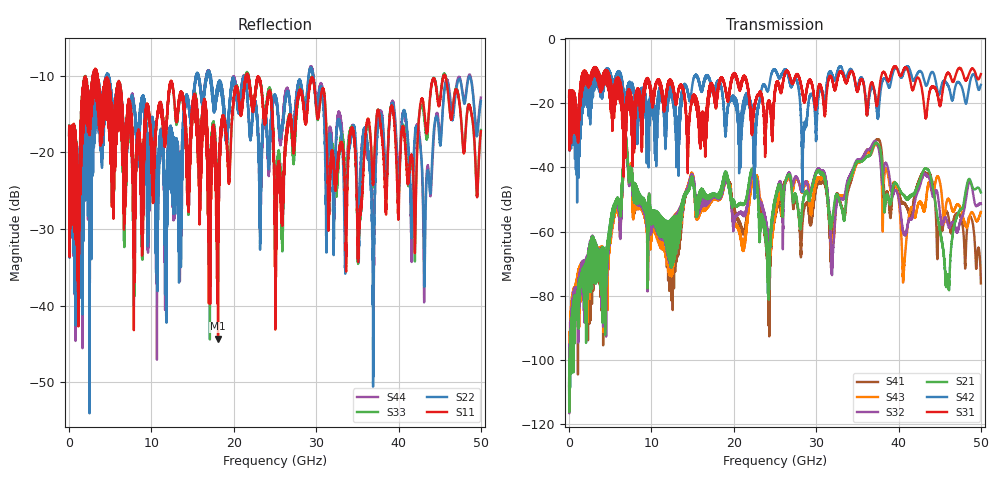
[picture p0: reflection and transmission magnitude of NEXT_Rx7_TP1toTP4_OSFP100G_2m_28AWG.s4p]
! Touchstone data
! Created: 27-Feb-2019 by IdEM 12 (12.1.0)
! COMMENTS
!  Created Wed Feb 27 12:03:36 2019
!  64 Port Network Data from SP1.SP block
!  freq  magS1_1  angS1_1  magS1_2  angS1_2  magS1_3  angS1_3  magS1_4  angS1_4
!  magS1_5  angS1_5  magS1_6  angS1_6  magS1_7  angS1_7  magS1_8  angS1_8
!  magS1_9  angS1_9  magS1_10  angS1_10  magS1_11  angS1_11  magS1_12  angS1_12
!  magS1_13  angS1_13  magS1_14  angS1_14  magS1_15  angS1_15  magS1_16  angS1_16
!  magS1_17  angS1_17  magS1_18  angS1_18  magS1_19  angS1_19  magS1_20  angS1_20
!  magS1_21  angS1_21  magS1_22  angS1_22  magS1_23  angS1_23  magS1_24  angS1_24
!  magS1_25  angS1_25  magS1_26  angS1_26  magS1_27  angS1_27  magS1_28  angS1_28
!  magS1_29  angS1_29  magS1_30  angS1_30  magS1_31  angS1_31  magS1_32  angS1_32
!  magS1_33  angS1_33  magS1_34  angS1_34  magS1_35  angS1_35  magS1_36  angS1_36
!  magS1_37  angS1_37  magS1_38  angS1_38  magS1_39  angS1_39  magS1_40  angS1_40
!  magS1_41  angS1_41  magS1_42  angS1_42  magS1_43  angS1_43  magS1_44  angS1_44
!  magS1_45  angS1_45  magS1_46  angS1_46  magS1_47  angS1_47  magS1_48  angS1_48
!  magS1_49  angS1_49  magS1_50  angS1_50  magS1_51  angS1_51  magS1_52  angS1_52
!  magS1_53  angS1_53  magS1_54  angS1_54  magS1_55  angS1_55  magS1_56  angS1_56
!  magS1_57  angS1_57  magS1_58  angS1_58  magS1_59  angS1_59  magS1_60  angS1_60
!  magS1_61  angS1_61  magS1_62  angS1_62  magS1_63  angS1_63  magS1_64  angS1_64
!  magS2_1  angS2_1  magS2_2  angS2_2  magS2_3  angS2_3  magS2_4  angS2_4
!  magS2_5  angS2_5  magS2_6  angS2_6  magS2_7  angS2_7  magS2_8  angS2_8
!  magS2_9  angS2_9  magS2_10  angS2_10  magS2_11  angS2_11  magS2_12  angS2_12
!  magS2_13  angS2_13  magS2_14  angS2_14  magS2_15  angS2_15  magS2_16  angS2_16
!  magS2_17  angS2_17  magS2_18  angS2_18  magS2_19  angS2_19  magS2_20  angS2_20
!  magS2_21  angS2_21  magS2_22  angS2_22  magS2_23  angS2_23  magS2_24  angS2_24
!  magS2_25  angS2_25  magS2_26  angS2_26  magS2_27  angS2_27  magS2_28  angS2_28
!  magS2_29  angS2_29  magS2_30  angS2_30  magS2_31  angS2_31  magS2_32  angS2_32
!  magS2_33  angS2_33  magS2_34  angS2_34  magS2_35  angS2_35  magS2_36  angS2_36
!  magS2_37  angS2_37  magS2_38  angS2_38  magS2_39  angS2_39  magS2_40  angS2_40
!  magS2_41  angS2_41  magS2_42  angS2_42  magS2_43  angS2_43  magS2_44  angS2_44
!  magS2_45  angS2_45  magS2_46  angS2_46  magS2_47  angS2_47  magS2_48  angS2_48
!  magS2_49  angS2_49  magS2_50  angS2_50  magS2_51  angS2_51  magS2_52  angS2_52
!  magS2_53  angS2_53  magS2_54  angS2_54  magS2_55  angS2_55  magS2_56  angS2_56
!  magS2_57  angS2_57  magS2_58  angS2_58  magS2_59  angS2_59  magS2_60  angS2_60
!  magS2_61  angS2_61  magS2_62  angS2_62  magS2_63  angS2_63  magS2_64  angS2_64
!  magS3_1  angS3_1  magS3_2  angS3_2  magS3_3  angS3_3  magS3_4  angS3_4
!  magS3_5  angS3_5  magS3_6  angS3_6  magS3_7  angS3_7  magS3_8  angS3_8
!  magS3_9  angS3_9  magS3_10  angS3_10  magS3_11  angS3_11  magS3_12  angS3_12
!  magS3_13  angS3_13  magS3_14  angS3_14  magS3_15  angS3_15  magS3_16  angS3_16
!  magS3_17  angS3_17  magS3_18  angS3_18  magS3_19  angS3_19  magS3_20  angS3_20
!  magS3_21  angS3_21  magS3_22  angS3_22  magS3_23  angS3_23  magS3_24  angS3_24
!  magS3_25  angS3_25  magS3_26  angS3_26  magS3_27  angS3_27  magS3_28  angS3_28
!  magS3_29  angS3_29  magS3_30  angS3_30  magS3_31  angS3_31  magS3_32  angS3_32
!  magS3_33  angS3_33  magS3_34  angS3_34  magS3_35  angS3_35  magS3_36  angS3_36
!  magS3_37  angS3_37  magS3_38  angS3_38  magS3_39  angS3_39  magS3_40  angS3_40
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# Hz S MA R 50
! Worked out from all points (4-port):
!   5000 points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, 10 MHz to 50 GHz, reference 50 ohm
!   strongest paths, dB at 10 MHz, 12.51 GHz, 25.01 GHz, 37.51 GHz, 50 GHz:
!     S31: -18.0, -14.0, -15.8, -18.9, -11.0
!     S42: -18.0, -16.4, -9.6, -24.1, -14.3
!     S21: -108.0, -64.5, -50.2, -32.7, -47.8
!     S32: -106.4, -64.6, -50.6, -33.4, -51.4
!     S43: -105.7, -63.4, -54.3, -33.5, -53.9
!     S41: -107.1, -64.1, -54.4, -31.4, -76.1
!   lowest |S11| = -44.3 dB at 18.09 GHz (marker M1), VSWR 1.01, Z = 49.5 + j0.362 ohm
!   |S11| at or under -10 dB: 3.49 GHz to 21.47 GHz (17.98 GHz wide, 144 % of centre); 21.77 GHz to 45.47 GHz (23.7 GHz wide, 70.5 % of centre); 45.66 GHz to end of sweep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
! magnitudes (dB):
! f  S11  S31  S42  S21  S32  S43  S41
! 10 MHz  -17.7  -18.0  -18.0  -108.0  -106.4  -105.7  -107.1
! 6.86 GHz  -26.8  -29.1  -24.4  -31.1  -32.6  -32.1  -30.6
! 18.09 GHz  -44.3  -16.7  -13.0  -49.2  -49.5  -49.5  -48.7
! 37.49 GHz  -14.5  -19.4  -24.9  -32.6  -33.2  -33.4  -31.3
! 40.64 GHz  -17.2  -9.4  -10.3  -48.6  -60.3  -71.8  -51.3
! 45.94 GHz  -11.6  -10.6  -14.3  -73.6  -57.2  -50.1  -54.1
! 50 GHz  -17.2  -11.0  -14.3  -47.8  -51.4  -53.9  -76.1
